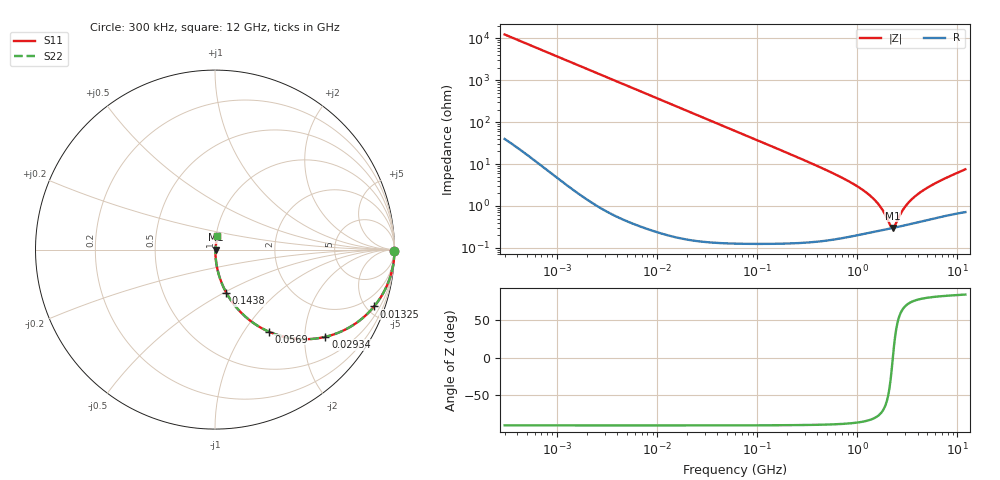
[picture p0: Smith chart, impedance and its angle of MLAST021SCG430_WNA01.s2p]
! MLAST021SCG430_WNA01  S-PARAMETER MODEL  ( Standard Model )
! Model Generated by TAIYO YUDEN Corporation (http://www.ty-top.com)
! Version 2.0
! TAIYO YUDEN Control No. 231201
! Copyright(c) 2023 TAIYO YUDEN CO.,LTD. All Rights Reserved.
! Product Description (link to TY-COMPAS)
! https://ds.yuden.co.jp/TYCOMPAS/or/detail?pn=MLAST021SCG430JWNA01&u=M
! Products Name : Multilayer Ceramic Capacitors
! Characteristics :
!  Capacitance : 43 [pF] , Rated Voltage : 25 [V] , TCC : CG / C0G
!  Case Size : 0.25 x 0.125 / 0.0098 x 0.0049 [mm/inch] , Thickness : 0.125 / 0.0049 [mm/inch]
!  (Conditions: Temperature = 25 [degC] , DC Bias Voltage = 0 [V])
! External Node Assignments :
!  1  o---| |---o  2
! GND o---------o GND
! Frequency Range : 0.3MHz  -  12000MHz  [ 401 STEP ]
# MHZ S RI R 50
! Freq[MHz].  S11 Real  S11 Imag  S21 Real  S21 Imag  S12 Real  S12 Imag  S22 Real  S22 Imag
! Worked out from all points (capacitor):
!   401 points, 300 kHz to 12 GHz, reference 50 ohm
!   read as one part in series: C = 43 pF near 316.3 kHz
!   lowest |Z| = 298 mohm at 2.261 GHz (marker M1)
!   series resonance near 2.261 GHz, so ESL is about 120 pH
!   S11 on the Smith chart (normalised r, x): 300 kHz: open; 13.25 MHz: 1.00, -5.60; 29.34 MHz: 1.00, -2.53; 56.9 MHz: 1.00, -1.30; 143.8 MHz: 1.00, -0.51; 12 GHz: 1.01, +0.15
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0.3  0.9999 -0.0081  9.17e-05 0.0081  9.17e-05 0.0081  0.9999 -0.0081
1.769972  0.9977 -0.0476  0.00231 0.0476  0.00231 0.0476  0.9977 -0.0476
4.716902  0.984 -0.1252  0.016 0.1252  0.016 0.1252  0.984 -0.1252
10.44266  0.9264 -0.2608  0.0736 0.2608  0.0736 0.2608  0.9264 -0.2608
13.25433  0.8866 -0.3168  0.1134 0.3168  0.1134 0.3168  0.8866 -0.3168
29.34352  0.6148 -0.4861  0.3852 0.4861  0.3852 0.4861  0.6148 -0.4861
56.90376  0.2982 -0.4565  0.7018 0.4565  0.7018 0.4565  0.2982 -0.4565
60  0.2765 -0.4463  0.7235 0.4463  0.7235 0.4463  0.2765 -0.4463
91.67136  0.141 -0.3465  0.859 0.3465  0.859 0.3465  0.141 -0.3465
143.8206  0.0628 -0.2402  0.9372 0.2402  0.9372 0.2402  0.0628 -0.2402
353.9943  0.0116 -0.1005  0.9884 0.1005  0.9884 0.1005  0.0116 -0.1005
763.2128  0.00355 -0.0423  0.9964 0.0423  0.9964 0.0423  0.00355 -0.0423
1229.528  0.00263 -0.0207  0.9974 0.0207  0.9974 0.0207  0.00263 -0.0207
1645.489  0.00265 -0.0102  0.9974 0.0102  0.9974 0.0102  0.00265 -0.0102
1829.429  0.00272 -0.00673  0.9973 0.00673  0.9973 0.00673  0.00272 -0.00673
2088.533  0.00286 -0.00249  0.9971 0.00249  0.9971 0.00249  0.00286 -0.00249
2261.293  0.00297 3.37e-06  0.997 -3.37e-06  0.997 -3.37e-06  0.00297 3.37e-06
2384.334  0.00306 0.00166  0.9969 -0.00166  0.9969 -0.00166  0.00306 0.00166
3026.31  0.00355 0.00915  0.9965 -0.00915  0.9965 -0.00915  0.00355 0.00915
3944.255  0.00433 0.0179  0.9957 -0.0179  0.9957 -0.0179  0.00433 0.0179
6188.031  0.0064 0.0353  0.9936 -0.0353  0.9936 -0.0353  0.0064 0.0353
12000  0.0125 0.0731  0.9875 -0.0731  0.9875 -0.0731  0.0125 0.0731
